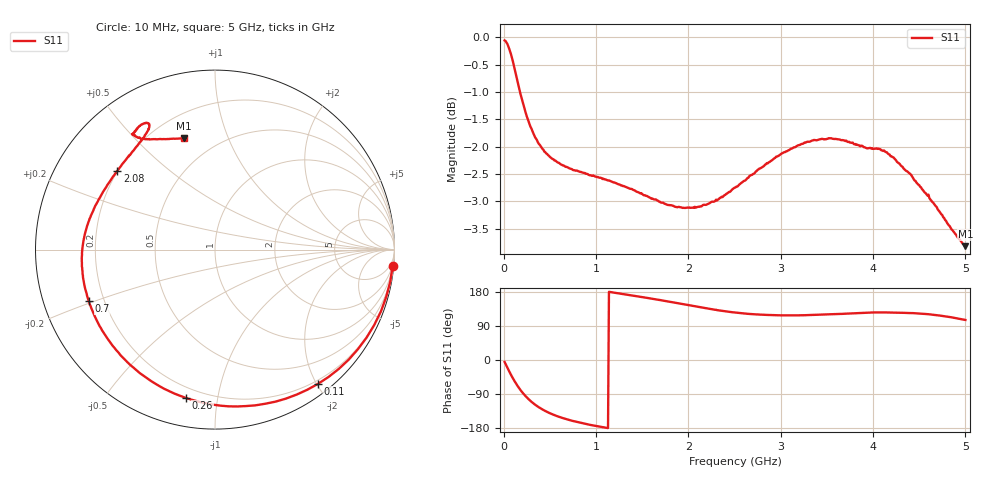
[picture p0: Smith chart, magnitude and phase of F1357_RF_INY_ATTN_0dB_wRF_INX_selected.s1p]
! S-parameters for RF_INY input IDT F1370 DPD Demodulator
! Date Measured:  2015-11-25  RGG
!  Port 1 = Pin 3 = RF_INY
! STATE: RF_INX selected, 0 dB attenuation (Gain = Gmax - 0 dB)
! RF Frequency:  10 MHz to 5000 MHz
! RF_INX, IF_I+, IF_I-, IF_Q+, and IF_Q- terminated
! 2300 MHz, 0 dBm signal applied to LO_IN
! Vcc = +5.00 Volts  Icc = approx 275 mA
! NOTES:  The device was measured on a custom printed circuit evaluation board with individual 50 ohm
!  microstrip lines to the RF and LO pins. The 50 ohm microstrip lines were de-embedded using reference
!  plane extensions
! Instrument Manufacturer:  Agilent Technologies
! Instrument Model:  E5071C
! Instrument Serial Number:  MY46419053
! Instrument Firmware Rev:  A.11.31
# HZ  S  RI R 50.00
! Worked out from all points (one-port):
!   500 points, 10 MHz to 5 GHz, reference 50 ohm
!   lowest |S11| = -3.8 dB at 5 GHz (marker M1), VSWR 4.62, Z = 16.6 + j35.2 ohm
!   |S11| at or under -10 dB: nowhere
!   S11 on the Smith chart (normalised r, x): 10 MHz: 1, -22; 110 MHz: 0.15, -2.02; 260 MHz: 0.14, -0.81; 700 MHz: 0.14, -0.19; 2.08 GHz: 0.20, +0.34; 5 GHz: 0.33, +0.70
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1e7  0.9896 -0.0911
3e7  0.9541 -0.2628
5e7  0.8868 -0.4208
8e7  0.7446 -0.6134
1.1e8  0.5728 -0.7485
1.4e8  0.3953 -0.8302
1.7e8  0.2267 -0.8675
2.1e8  0.0318 -0.8697
2.6e8  -0.1622 -0.8264
3.3e8  -0.3572 -0.7315
4.1e8  -0.5001 -0.615
5.1e8  -0.6072 -0.4837
6.4e8  -0.6818 -0.3437
7e8  -0.703 -0.2885
9.4e8  -0.7394 -0.1123
1.26e9  -0.7306 0.061
1.57e9  -0.684 0.2066
1.89e9  -0.6028 0.355
2.08e9  -0.5437 0.4384
2.51e9  -0.4207 0.5952
2.82e9  -0.371 0.6665
3.13e9  -0.3692 0.7006
3.43e9  -0.3976 0.7021
3.76e9  -0.4342 0.6732
4.06e9  -0.4602 0.6434
4.38e9  -0.4212 0.6238
4.68e9  -0.3351 0.6153
5e9  -0.1737 0.6201
